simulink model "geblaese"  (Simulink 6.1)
settings: Solver=FixedStepDiscrete  StartTime=0.0  StopTime=100  FixedStep=0.0001  RelTol=1e-3
libraries: simulink x2

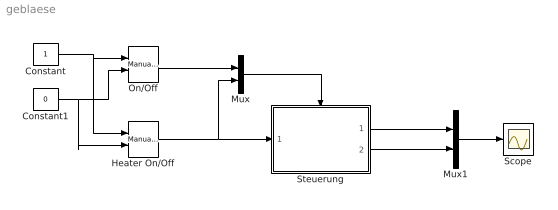
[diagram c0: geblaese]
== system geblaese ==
  Constant : Constant
  Constant1 : Constant  Value=0
  Heater On/Off : simulink/Signal Routing/Manual Switch  sw=0  action=0
  Mux : Mux  Inputs=2
  Mux1 : Mux  Inputs=2
  On/Off : simulink/Signal Routing/Manual Switch  sw=0  action=0
  Scope : Scope
  Steuerung : Stateflow chart  TreatAsAtomicUnit=on
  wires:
  Constant1/1 -> On/Off/2, Heater On/Off/2
  Constant/1 -> On/Off/1, Heater On/Off/1
  Mux/1 -> Steuerung/Trigger
  On/Off/1 -> Mux/1
  Heater On/Off/1 -> Mux/2, Steuerung/1(heater)
  Steuerung/1(fan_on) -> Mux1/1
  Steuerung/2(heat_on) -> Mux1/2
  Mux1/1 -> Scope/1

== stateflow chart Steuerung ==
  state Fan [parallel]
    state On/
      en:fan_on=1;
    state Off/
      en: fan_on=0;
    (default) -> Off
    Off -> On : SwFan
    On -> Off : SwFan/HeaterOff;
  state Heater [parallel]
    state Off/
      en:heat_on=0;
    state On/
      en:heat_on=1;
    Off -> On : [in(Fan.On) && heater==1]
    On -> Off : SwHeater | HeaterOff
    (default) -> Off
